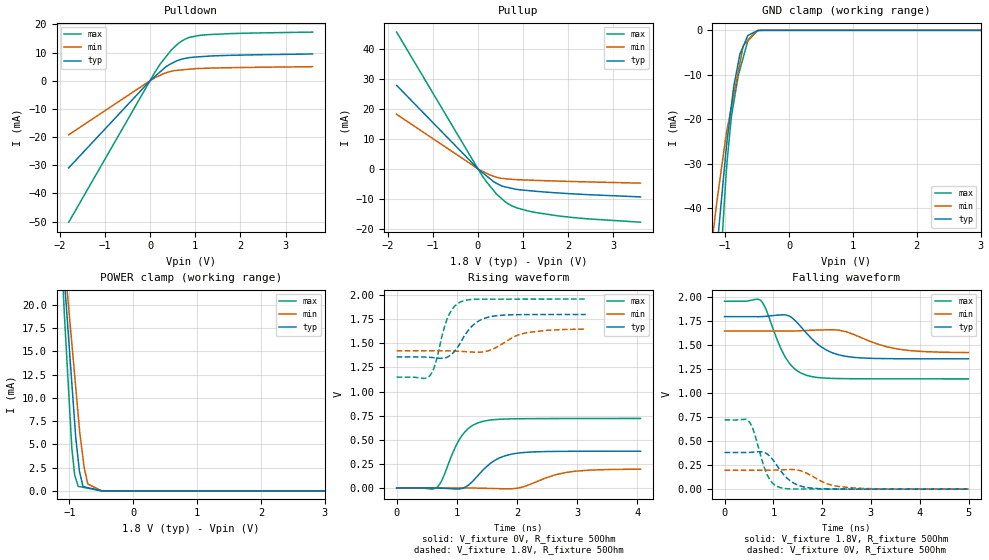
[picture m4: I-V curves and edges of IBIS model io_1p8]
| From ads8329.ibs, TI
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|   io_1p8 Model
[Model]   io_1p8
Model_type   I/O
Polarity   Non-Inverting
Enable   Active-Low
Vinl = 0.63
Vinh = 1.17
Vmeas = 0.9
Vref = 0.9
Cref = 30pF
Rref = 50
|   typ   min   max
|   (nom PVT)   (Fast PVT)   (slow PVT)
|C_comp from frequency sweep method(F=50MHz)
|Average
C_comp   4.252e-12   4.173e-12   4.361e-12
|C_comp   4.136e-12   4.036e-12   4.247e-12
|ON state : BUFFER OUTPUT TURNED HIGH
|C_comp   4.252e-12   4.173e-12   4.361e-12
|OFF state: BUFFER OUTPUT TURNED LOW
|C_comp   4.020e-12   3.900e-12   4.134e-12
|C_comp from LC tank measurement(L=1nH)
|C_comp   2.970e+09   3.090e+09   2.840e+09
|OFF state: BUFFER OUTPUT TURNED LOW
|Resonant Frequency(Hz)   2.970e+09   3.090e+09   2.840e+09
|C_comp   2.874e-12   2.656e-12   3.144e-12
|ON state : BUFFER OUTPUT TURNED HIGH
|Resonant Frequency(Hz)   2.930e+09   3.070e+09   2.760e+09
|C_comp   2.953e-12   2.690e-12   3.329e-12
| Where nom  PVT is Nominal Process,  1.8V,  28C
|   Fast PVT is Strong Process,   1.96V, -40C
|   Slow PVT is Weak Process,   1.65V,  88C
[Model Spec]
Vinl   0.63   0.58   0.68
Vinh   1.17   1.07   1.27
[Voltage Range]   1.8   1.65   1.96
|Ambient Temperature   25   85   -40
|Junction Temperature
[Temperature Range]   28   88   -40
[Pullup Reference]   1.8   1.65   1.96
[Pulldown Reference]   0   0   0
[Power Clamp Reference]   1.8   1.65   1.96
[GND Clamp Reference]   0   0   0
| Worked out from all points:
|   slope of the pulldown table from 0 to 0.27 V, typ, clamps not added: 70.5 ohm
|   slope of the pullup table from 0 to 0.27 V, typ, clamps not added: 81.1 ohm
|   GND clamp passes 1 mA (typ) near -0.62 V on its own axis
|   POWER clamp passes 1 mA (typ) near -0.80 V on its own axis
|   falling waveform, V_fixture 1.8V, R_fixture 50Ohm: 20-80 % time 569ps typ, 781ps min, 426ps max; typ from 1.8 V to 1.36 V
|   rising waveform, V_fixture 0V, R_fixture 50Ohm: 20-80 % time 413ps typ, 554ps min, 332ps max; typ from 0 V to 0.382 V
|   rising waveform, V_fixture 1.8V, R_fixture 50Ohm: 20-80 % time 316ps typ, 423ps min, 217ps max; typ from 1.36 V to 1.8 V
|   falling waveform, V_fixture 0V, R_fixture 50Ohm: 20-80 % time 387ps typ, 493ps min, 264ps max; typ from 0.383 V to 0 V
[Pulldown]
|   Voltage   I(typ)   I(min)   I(max)
-1.8V     -30.93mA   -19.17mA   -50.22mA
0V        0A         0A         0A
96.04mV   1.385mA    924.7uA    2.686mA
235.2mV   3.339mA    2.047mA    6.166mA
349.2mV   4.939mA    2.816mA    8.461mA
470.4mV   6.1mA      3.378mA    10.9mA
617.4mV   7.24mA     3.735mA    13.1mA
705.6mV   7.698mA    3.866mA    14.13mA
852.6mV   8.181mA    4.085mA    15.3mA
1.188V    8.631mA    4.421mA    16.27mA
1.776V    9.033mA    4.643mA    16.75mA
3.6V      9.519mA    5.015mA    17.29mA
[GND Clamp]
|   Voltage   I(typ)   I(min)   I(max)
-1.8V     -179.7mA   -127.6mA   -265.7mA
-1.277V   -75.61mA   -56.26mA   -107.5mA
-1.129V   -49.2mA    -38.47mA   -66.75mA
-1.113V   -46.82mA   -36.88mA   -62.55mA
-990mV    -27.62mA   -24.08mA   -33.51mA
-903.6mV  -17.09mA   -17.36mA   -19.55mA
-865.8mV  -12.68mA   -14.56mA   -16.28mA
-768.6mV  -5.385mA   -7.369mA   -8.837mA
-714.5mV  -3.531mA   -3.361mA   -6.002mA
-644.4mV  -1.177mA   -2.331mA   -2.335mA
-456.7mV  -16.48uA   -17.11uA   -14.45uA
3.6V      0A         0A         0A
[Pullup]
|   Voltage   I(typ)   I(min)   I(max)
-1.8V     27.83mA    18.17mA    45.6mA
0V        0A         0A         0A
96.04mV   -1.206mA   -771.1uA   -2.301mA
180.3mV   -2.235mA   -1.414mA   -4.157mA
407.7mV   -4.805mA   -2.758mA   -8.363mA
599.8mV   -6.008mA   -3.29mA    -10.95mA
852.6mV   -6.865mA   -3.612mA   -12.97mA
1.272V    -7.471mA   -3.851mA   -14.56mA
2.111V    -8.348mA   -4.237mA   -16.25mA
3.6V      -9.363mA   -4.766mA   -17.8mA
[POWER Clamp]
|   Voltage   I(typ)   I(min)   I(max)
-1.8V     100.6mA    87.75mA    118.7mA
-1.092V   24.73mA    26.07mA    21.2mA
-1.06V    21.14mA    23.59mA    16.88mA
-958.4mV  11.41mA    15.72mA    4.466mA
-915.3mV  7.285mA    12.38mA    1.69mA
-896.4mV  5.545mA    10.92mA    1.275mA
-860.4mV  3.311mA    8.134mA    485.6uA
-840.6mV  2.079mA    6.599mA    459.8uA
-784.8mV  468.3uA    3.455mA    387uA
-709.5mV  348.9uA    734.4uA    288.8uA
-488.4mV  49.53nA    1.027uA    472.7nA
3.6V      0A         0A         0A
[Ramp]
R_load = 50
|   typ   min   max
dV/dt_r   0.229407/4.13062e-10   0.117986/5.55648e-10   0.433168/3.31918e-10
dV/dt_f   0.2642/5.67739e-10   0.134982/7.71695e-10   0.485804/4.2597e-10
[Falling Waveform]
V_fixture = 1.8V
V_fixture_min = 1.65V
V_fixture_max = 1.96V
R_fixture = 50Ohm
|   Time   V(typ)   V(min)   V(max)
0s        1.8V       1.65V      1.96V
740ps     1.8V       1.65V      1.97V
844ps     1.803V     1.65V      1.882V
1.256ns   1.816V     1.649V     1.368V
1.448ns   1.757V     1.651V     1.251V
1.678ns   1.628V     1.656V     1.188V
2.082ns   1.453V     1.662V     1.158V
2.5ns     1.385V     1.641V     1.153V
3.532ns   1.361V     1.463V     1.151V
4.998ns   1.36V      1.425V     1.15V
[Rising Waveform]
V_fixture = 0V
V_fixture_min = 0V
V_fixture_max = 0V
R_fixture = 50Ohm
|   Time   V(typ)   V(min)   V(max)
0s        776.7pV    893pV      637.9pV
664ps     193.5uV    122.8uV    4.077mV
756ps     -1.527mV   207.2uV    84.18mV
950ps     -8.685mV   389uV      387.6mV
1.082ns   -4.254mV   493.4uV    539.8mV
1.428ns   181.5mV    -2.027mV   690.3mV
1.704ns   310.5mV    -6.502mV   712.8mV
2.024ns   362.4mV    723uV      718.4mV
2.812ns   380.6mV    160.8mV    720.7mV
4.056ns   382.1mV    195.6mV    721.6mV
[Rising Waveform]
V_fixture = 1.8V
V_fixture_min = 1.65V
V_fixture_max = 1.96V
R_fixture = 50Ohm
|   Time   V(typ)   V(min)   V(max)
0s        1.359V     1.423V     1.15V
550ps     1.356V     1.424V     1.164V
642ps     1.35V      1.424V     1.286V
844ps     1.358V     1.423V     1.759V
952ps     1.41V      1.421V     1.877V
1.08ns    1.526V     1.417V     1.934V
1.276ns   1.693V     1.409V     1.957V
1.532ns   1.773V     1.425V     1.959V
2.118ns   1.798V     1.604V     1.959V
3.146ns   1.8V       1.648V     1.959V
[Falling Waveform]
V_fixture = 0V
V_fixture_min = 0V
V_fixture_max = 0V
R_fixture = 50Ohm
|   Time   V(typ)   V(min)   V(max)
0s        383mV      197.2mV    722.7mV
512ps     384.2mV    196.9mV    699.4mV
608ps     387.1mV    196.8mV    588.4mV
876ps     365.9mV    197.6mV    147.8mV
1.15ns    192mV      201.4mV    15.04mV
1.398ns   69.52mV    205.4mV    2.623mV
1.724ns   14.62mV    156.4mV    1.661mV
2.138ns   2.817mV    49.79mV    1.297mV
2.588ns   1.124mV    14.92mV    1.009mV
4.998ns   366uV      323.3uV    406.2uV
